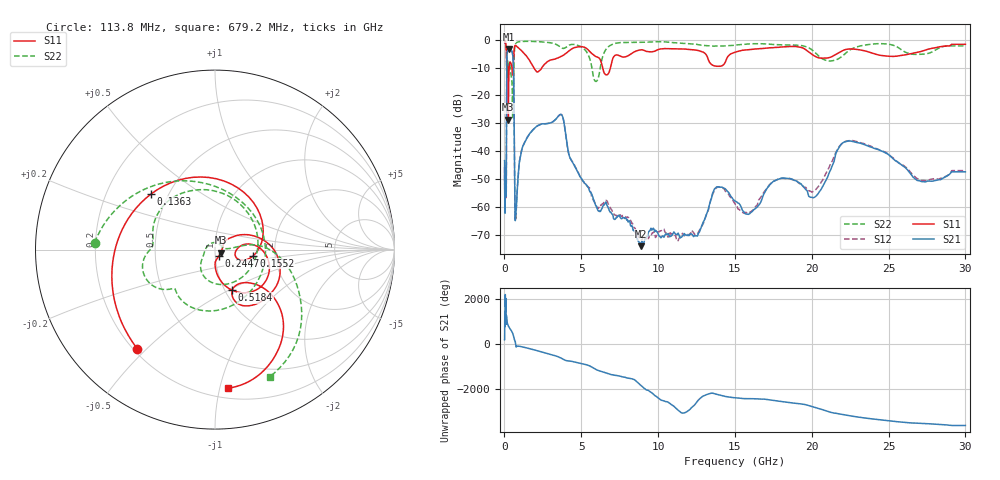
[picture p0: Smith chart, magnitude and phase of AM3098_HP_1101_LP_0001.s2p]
! Date/Time: Thu, Feb 28, 2019 8:45 AM
! Network Analyzer: Agilent Technologies E8364B Rev: A.07.50.67
! Sweep from 0.010 to 30.000 GHz, 1601 Points, Sweep Type: LOG
! Power Supply: 5.022 V, 0.002 A
# Hz S DB R 50
!freq MagS11 AngS11 MagS21 AngS21 MagS12 AngS12 MagS22 AngS22
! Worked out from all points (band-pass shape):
!   1601 points, 10 MHz to 30 GHz, reference 50 ohm
!   highest |S21| = -3.33 dB at 266.5 MHz (marker M1); lowest = -74.0 dB at 8.893 GHz (marker M2)
!   |S21| within 3 dB of the highest: 158.7 MHz to 551.4 MHz (392.7 MHz wide, 111 % of centre)
!   lowest |S11| = -28.7 dB at 249.7 MHz (marker M3), VSWR 1.08, Z = 53.3 - j1.85 ohm
!   |S11| at or under -10 dB: 206.3 MHz to 306.4 MHz (100.1 MHz wide, 39.1 % of centre); 1.898 GHz to 2.438 GHz (540.1 MHz wide, 24.9 % of centre); 6.382 GHz to 6.902 GHz (520.3 MHz wide, 7.83 % of centre)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
!   |S22| runs from -28.3 to -0.5 dB; largest |S21 - S12| = 0.011
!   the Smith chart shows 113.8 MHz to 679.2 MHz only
!   S11 on the Smith chart (normalised r, x): 113.8 MHz: 0.22, -0.47; 136.3 MHz: 0.40, +0.32; 155.2 MHz: 1.54, -0.11; 244.7 MHz: 1.04, -0.08; 518.4 MHz: 1.08, -0.52; 679.2 MHz: 0.27, -1.06
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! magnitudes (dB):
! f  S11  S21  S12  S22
! 10 MHz  -0.3  -43.4  -47.3  -0.6
! 38.04 MHz  -0.3  -60.9  -57.3  -0.6
! 113.8 MHz  -3.1  -52.4  -55.6  -3.5
! 136.3 MHz  -6.5  -25.8  -25.7  -10.5
! 144.7 MHz  -8.7  -14.2  -14.1  -10.2
! 155.2 MHz  -13.3  -7.3  -7.3  -9.5
! 208.5 MHz  -10.3  -3.9  -3.9  -7.7
! 244.7 MHz  -27.5  -3.4  -3.4  -9.1
! 249.7 MHz  -28.7  -3.4  -3.3  -9.1
! 266.5 MHz  -18.9  -3.3  -3.3  -9.2
! 518.4 MHz  -12.2  -4.9  -4.8  -24.4
! 550.5 MHz  -12.2  -6.3  -6.2  -28.0
! 605.4 MHz  -5.7  -15.6  -15.5  -11.6
! 679.2 MHz  -2.2  -59.8  -59.0  -2.3
! 2.084 GHz  -11.5  -31.1  -31.2  -0.7
! 3.704 GHz  -6.0  -26.8  -26.9  -2.9
! 5.959 GHz  -6.1  -59.5  -59.3  -15.0
! 7.926 GHz  -6.1  -64.3  -63.7  -1.0
! 8.893 GHz  -3.7  -74.0  -71.6  -1.0
! 20.2 GHz  -5.9  -56.4  -54.1  -4.6
! 22.56 GHz  -3.3  -36.4  -36.2  -3.5
! 30 GHz  -1.7  -47.4  -46.9  -2.3
